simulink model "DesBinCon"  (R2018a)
settings: Solver=VariableStepAuto  StartTime=0.0  StopTime=10  RelTol=1e-3
undefined symbols (not defined in the file): d003cc01, DesBinCon, sdiscope

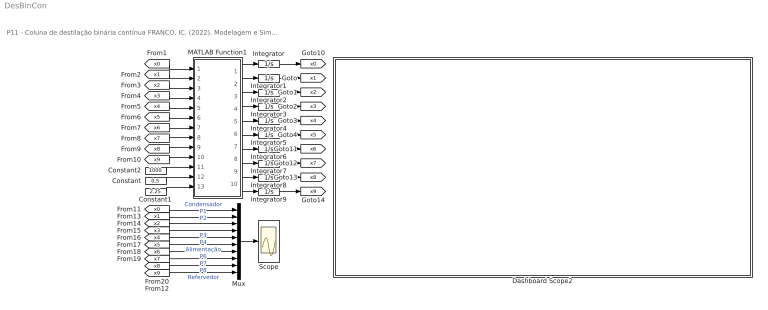
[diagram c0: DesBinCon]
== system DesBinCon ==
  note: P11 - Coluna de destilação binária contínua FRANCO, IC. (2022). Modelagem e Simulação: Problemas Típicos da Engenharia Química para Simulação e Análise. NOTAS DE AULA INOVADORAS. The Journal of Engineering and Exact Sciences. Material Complementar.
  Constant : Constant  Value=0.5
  Constant1 : Constant  Value=2.25
  Constant2 : Constant  Value=1000
  Dashboard Scope2 : Subsystem  DialogController=hmiCreateDDGDialog  IsWebBlock=on  mask(MWDashboardBlock){webBlockId=d003cc01-33f6-444b-9fc2-2e99a7f36cc5, webBlockType=sdiscope, ShowInitialText=on, HMISrcModelName=DesBinCon}
      mask prompts: webBlockId "WebBlock Id"; webBlockType "WebBlock Type"; HMISrcModelName "Source Model"
      mask help: SimulinkHMI:dialogs:HMIScopeDialogDesc
  Integrator{,1..9} (10 alike) : Integrator
  MATLAB Function1 : MATLAB Function  TreatAsAtomicUnit=on
  Mux : Mux  Inputs=10
  Scope : Scope
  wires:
  Constant/1 -> MATLAB Function1/12(x)
  Constant2/1 -> MATLAB Function1/11(F)
  MATLAB Function1/1(dx0) -> Integrator/1
  Integrator/1 -> [x0]
  [x0] -> MATLAB Function1/1(x0)
  MATLAB Function1/2(dx1) -> Integrator1/1
  Integrator1/1 -> [x1]
  [x1] -> MATLAB Function1/2(x1)
  [x2] -> MATLAB Function1/3(x2)
  MATLAB Function1/3(dx2) -> Integrator2/1
  Integrator2/1 -> [x2]
  [x3] -> MATLAB Function1/4(x3)
  MATLAB Function1/4(dx3) -> Integrator3/1
  Integrator3/1 -> [x3]
  MATLAB Function1/5(dx4) -> Integrator4/1
  Integrator4/1 -> [x4]
  [x4] -> MATLAB Function1/5(x4)
  MATLAB Function1/6(dx5) -> Integrator5/1
  Integrator5/1 -> [x5]
  [x5] -> MATLAB Function1/6(x5)
  MATLAB Function1/7(dx6) -> Integrator6/1
  Integrator6/1 -> [x6]
  [x6] -> MATLAB Function1/7(x6)
  MATLAB Function1/8(dx7) -> Integrator7/1
  [x7] -> MATLAB Function1/8(x7)
  Integrator7/1 -> [x7]
  MATLAB Function1/9(dx8) -> Integrator8/1
  Integrator8/1 -> [x8]
  [x8] -> MATLAB Function1/9(x8)
  Integrator9/1 -> [x9]
  MATLAB Function1/10(dx9) -> Integrator9/1
  [x9] -> MATLAB Function1/10(x9)
  Constant1/1 -> MATLAB Function1/13(R)
  [x3] -> Mux/4  "P3"
  [x5] -> Mux/6  "Alimentação"
  [x8] -> Mux/9  "P8"
  [x2] -> Mux/3  "P2"
  [x9] -> Mux/10  "Refervedor"
  [x0] -> Mux/1  "Condensador"
  [x7] -> Mux/8  "P7"
  [x6] -> Mux/7  "P6"
  [x1] -> Mux/2  "P1"
  [x4] -> Mux/5  "P4"
  Mux/1 -> Scope/1

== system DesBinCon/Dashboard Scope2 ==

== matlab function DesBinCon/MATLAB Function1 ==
function [dx0,dx1,dx2,dx3,dx4,dx5,dx6,dx7,dx8,dx9]=fcn(x0,x1,x2,x3,x4,x5,x6,x7,x8,x9,F,x,R)
%% Parâmetros
M0    =  200.00;
MP    =   50.00;
MR    =  400.00;
q     =    1.00;
VL    = 1575.00;
alpha =    2.46;

%% equações auxiliares
% vazões molares
V  = VL-(1-q)*F;
D  = V/(R+1);
L  = R*D;
LL = F+q*F;
W  = LL-VL;

% equilíbrio líquido-vapor
y1=alpha*x1/(1+(alpha-1)*x1);
y2=alpha*x2/(1+(alpha-1)*x2);
y3=alpha*x3/(1+(alpha-1)*x3);
y4=alpha*x4/(1+(alpha-1)*x4);
y5=alpha*x5/(1+(alpha-1)*x5);
y6=alpha*x6/(1+(alpha-1)*x6);
y7=alpha*x7/(1+(alpha-1)*x7);
y8=alpha*x8/(1+(alpha-1)*x8);
y9=alpha*x9/(1+(alpha-1)*x9);

%% Modelo matemático
dx0=(1/M0)*(V*y1-(L+D)*x0);
dx1=(1/MP)*(L*(x0-x1)+V*(y2-y1));
dx2=(1/MP)*(L*(x1-x2)+V*(y3-y2));
dx3=(1/MP)*(L*(x2-x3)+V*(y4-y3));
dx4=(1/MP)*(L*(x3-x4)+V*(y5-y4));
dx5=(1/MP)*(L*x4-LL*x5+VL*y6-V*y5+F*x);
dx6=(1/MP)*(LL*(x5-x6)+VL*(y7-y6));
dx7=(1/MP)*(LL*(x6-x7)+VL*(y8-y7));
dx8=(1/MP)*(LL*(x7-x8)+VL*(y9-y8));
dx9=(1/MR)*(LL*x8-W*x9-VL*y9);
end
